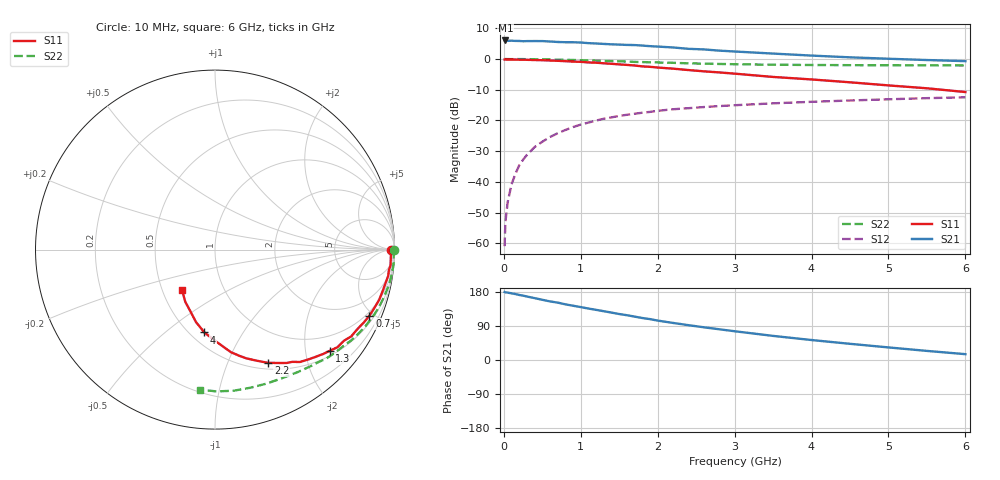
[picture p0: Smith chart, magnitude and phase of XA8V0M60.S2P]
! SIEMENS Discrete & RF Semiconductors
! BFY180
! Si NPN RF Bipolar Junction Transistor in MICRO-X
! VCE = 8 V  IC = 0.6 mA
! Common Emitter S-Parameters:  May  1997
# GHz  S  MA  R  50
!  f  S11  S21  S12  S22
! GHz  MAG  ANG  MAG  ANG  MAG  ANG  MAG  ANG
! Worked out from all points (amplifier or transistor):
!   36 points, 10 MHz to 6 GHz, reference 50 ohm
!   highest |S21| = 6.0 dB at 20 MHz (marker M1)
!   |S21| within 3 dB of that: start of sweep to 2.643 GHz
!   unconditionally stable (mu >= 1): 5.73 GHz to end of sweep
!   at 250 MHz: K = 0.06, MSG = 19.3 dB, |S12| = -32.8 dB
!   at 1.4 GHz: K = 0.40, MSG = 11.9 dB, |S12| = -19.0 dB
!   at 6 GHz: K = 1.01, MAG = 5.2 dB, |S12| = -12.5 dB
!   S11 on the Smith chart (normalised r, x): 10 MHz: open; 700 MHz: 0.80, -4.74; 1.3 GHz: 0.61, -2.51; 2.2 GHz: 0.58, -1.41; 4 GHz: 0.59, -0.69; 6 GHz: 0.63, -0.31
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0.01  0.9808 -0.2  1.984 179.4  0.0009 85.7  0.9978 -0.1
0.02  0.9873 -0.7  2.006 178.6  0.0022 97.9  0.9999 -0.4
0.05  0.9803 -1.5  1.975 177.9  0.0047 83.9  0.9976 -1.1
0.1  0.9809 -3.4  1.988 175.9  0.0091 88.4  0.9958 -2.3
0.2  0.9756 -6.6  1.968 171.6  0.0186 86.4  0.9975 -4.6
0.3  0.9713 -10.0  1.958 167.5  0.0275 82.6  0.9947 -6.9
0.4  0.9631 -13.5  1.962 163.3  0.0369 79.8  0.9928 -9.2
0.6  0.9461 -20.0  1.929 154.6  0.0538 74.6  0.9826 -13.7
0.7  0.9361 -23.2  1.895 151.4  0.062 72.2  0.9773 -15.9
0.9  0.9079 -29.4  1.876 143.2  0.0781 67.2  0.9645 -20.3
1.1  0.8801 -35.2  1.814 135.8  0.0925 62.5  0.9492 -24.4
1.3  0.8521 -41.5  1.762 128.7  0.1067 58.1  0.9339 -28.5
1.7  0.7848 -52.9  1.688 114.5  0.1287 50.3  0.8983 -36.0
2  0.7272 -60.3  1.595 104.0  0.1436 45.2  0.8794 -41.1
2.2  0.6974 -64.8  1.543 97.8  0.1523 41.7  0.8677 -44.5
2.6  0.6306 -73.9  1.434 86.3  0.1654 36.2  0.8415 -50.3
2.8  0.6056 -77.3  1.37 81.1  0.1715 33.8  0.8315 -53.1
3.5  0.511 -89.5  1.227 63.6  0.1901 25.9  0.8082 -62.4
4  0.4655 -97.3  1.138 52.7  0.2013 20.9  0.7999 -69.0
4.5  0.418 -104.6  1.066 42.7  0.2115 16.4  0.7944 -75.6
5.5  0.334 -119.8  0.963 24.0  0.2309 7.4  0.7902 -89.4
6  0.2903 -129.2  0.924 15.4  0.2383 2.8  0.7844 -96.3
